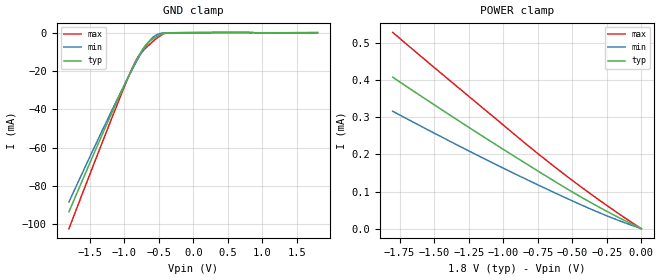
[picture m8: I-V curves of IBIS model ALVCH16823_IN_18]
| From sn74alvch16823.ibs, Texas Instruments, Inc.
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[Model]   ALVCH16823_IN_18
Model_type  Input
Vinl=0.5775
Vinh=1.2675
| variable   typ   min   max
C_comp   2.71pF   2.07pF   3.19pF
[Temperature Range]   40   100   -40
| Ambient temperature   25   85   -40
[Voltage range]   1.8   1.65   1.95
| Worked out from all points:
|   GND clamp passes 1 mA (typ) near -0.47 V on its own axis
[GND Clamp]
| ALVCH16823_IN_18
|   Voltage   I(typ)   I(min)   I(max)
-1.8V     -93.39mA   -88.25mA   -102.2mA
-1.235V   -46.33mA   -44.77mA   -49.66mA
-1V       -27.56mA   -27.45mA   -28.45mA
-875mV    -18.1mA    -18.66mA   -17.83mA
-795mV    -12.51mA   -13.33mA   -12.44mA
-700mV    -7.041mA   -7.586mA   -8.484mA
-615mV    -4.026mA   -3.532mA   -5.571mA
-540mV    -2.292mA   -1.342mA   -3.273mA
-445mV    -581uA     -184.1uA   -947.9uA
-375mV    -76.18uA   -61.83uA   -109.3uA
1.8V      25.63pA    20.14uA    -34.81uA
[POWER Clamp]
| ALVCH16823_IN_18
|   Voltage   I(typ)   I(min)   I(max)
-1.8V     408uA      316.3uA    528.6uA
-1.19V    258.8uA    198.3uA    338.2uA
-685mV    140.6uA    106.7uA    183.3uA
-335mV    63.93uA    47.84uA    85.01uA
-16.28fV  25.63pA    130.8pA    27.64pA
